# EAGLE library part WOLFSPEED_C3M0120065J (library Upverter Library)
Silicon Carbide Power MOSFET N-Channel 650 V 21A (Tc) 86W (Tc) RDS(on) 120mohm
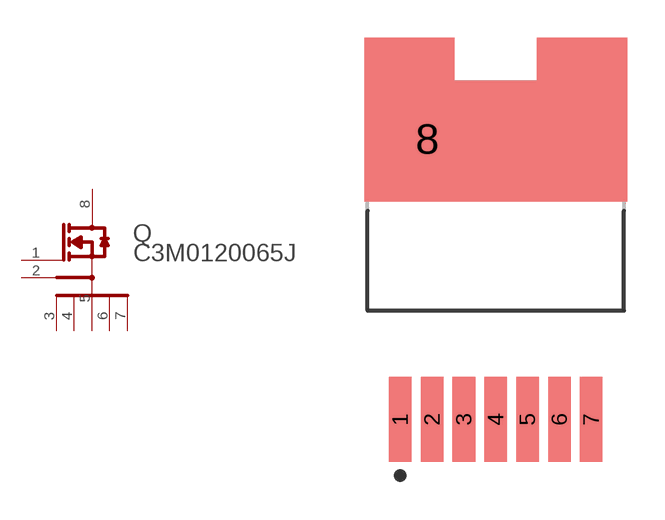
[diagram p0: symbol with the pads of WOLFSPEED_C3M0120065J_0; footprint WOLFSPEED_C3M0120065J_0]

Designator prefix Q

## WOLFSPEED_C3M0120065JWOLFSPEED_C3M0120065J_0_0 (MF: Wolfspeed; MPN: C3M0120065J; automotive: No; centroid_not_specified: Yes; continuous_drain_current: 21A; datasheet: https://assets.wolfspeed.com/uploads/2021/05/C3M0120065J.pdf; depletion_mode: False; device_class_L1: Discrete Semiconductors; device_class_L2: Transistors; device_class_L3: MOSFETs; digikey_description: 650V 120M SIC MOSFET; digikey_part_number: 1697-C3M0120065J-ND; drain_to_source_breakdown_voltage: 650V; drain_to_source_resistance: 120mΩ; drain_to_source_voltage: 650V; footprint_variant_name_0: Recommended_Land_Pattern; gate_charge_at_vgs: 26nC @ 15V; gate_to_source_voltage: 19V; height: 4.82mm; input_capacitace_at_vds: 640pF @ 400V; lead_free: Yes; max_junction_temp: +175°C; mfg_package_ident: TO-263-7; mfg_package_ident_component_id: d2de6d38281de76c; mfg_package_ident_date: 0; mfg_package_ident_rev: 0; mouser_part_number: 941-C3M0120065J; number_of_N_channels: 1; number_of_channels: 1; package: TO-263-7; power_dissipation: 86W; prefix: Q; pulse_drain_current: 51A; reverse_recovery_charge: 78nC; reverse_recovery_time: 8ns; rohs: Yes; rthja_max: 40°C/W; standoff_height: 0mm; technology: SiC; temperature_range_high: +175°C; temperature_range_low: -40°C; threshold_vgs_max: 3.6V; threshold_vgs_min: 1.8V; transconductance: 5S; turn_off_delay_time: 18ns; turn_on_delay_time: 8ns; typ_forward_diode_voltage: 4.5V; verification_version: 0.0.0.3)  [WOLFSPEED_C3M0120065J_0]
1  GATE  pas
2  DRIVER_SOURCE  pas
3  1_POWER_SOURCE  pas
4  2_POWER_SOURCE  pas
5  3_POWER_SOURCE  pas
6  4_POWER_SOURCE  pas
7  5_POWER_SOURCE  pas
8  DRAIN  pas

## Footprint WOLFSPEED_C3M0120065J_0 (pad centres in mm)
Silicon Carbide Power MOSFET N-Channel 650 V 21A (Tc) 86W (Tc) RDS(on) 120mohm
smd 0.9 x 3.4: 1 -3.81,-6.764; 2 -2.54,-6.764; 3 -1.27,-6.764; 4 0,-6.764; 5 1.27,-6.764; 6 2.54,-6.764; 7 3.81,-6.764
smd 4.505 x 4.505: 8 -2.737,4.429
